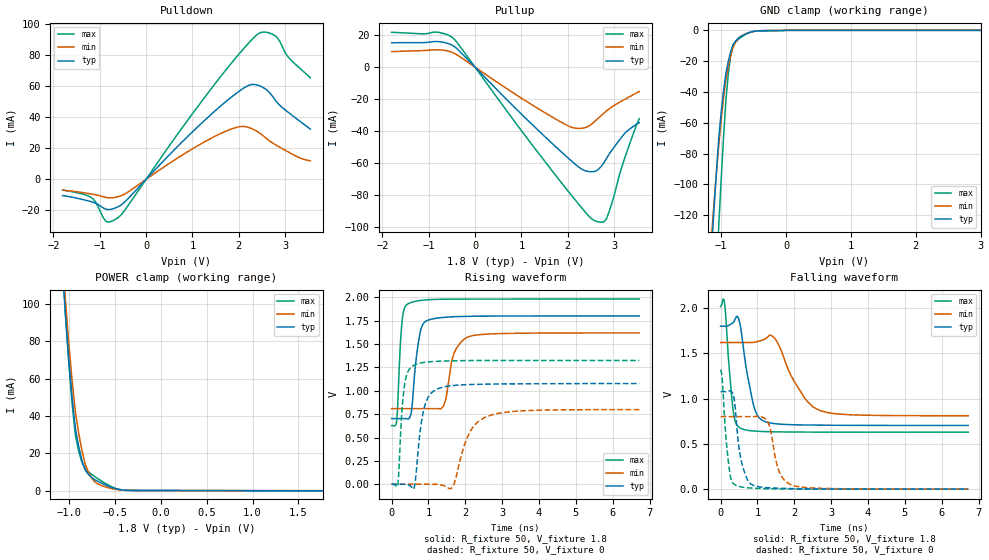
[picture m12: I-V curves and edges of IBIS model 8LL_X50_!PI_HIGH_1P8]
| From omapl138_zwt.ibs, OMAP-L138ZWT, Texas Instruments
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|   Model Cell 8LL_X50_!PI_HIGH_1P8
|BC1833DV40CTPBFZ_!PI_HIGH_1P8
[Model]   8LL_X50_!PI_HIGH_1P8
Model_type   I/O
Polarity   Non-Inverting
Enable   Active-Low
Vinl =  0.63
Vinh =  1.17
Cref =  15pF
Rref =  100.00M
Vref =  0V
Vmeas =  0.9
C_comp   2.232809p   2.073051p   2.295852p
[Model Spec]
Vinl   0.63   0.567   0.693
Vinh   1.17   1.053   1.287
[Temperature Range]   25   125   -40
[Voltage Range]   1.8   1.62   1.98
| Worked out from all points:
|   slope of the pulldown table from 0 to 0.27 V, typ, clamps not added: 31.4 ohm
|   slope of the pullup table from 0 to 0.27 V, typ, clamps not added: 33.4 ohm
|   GND clamp passes 1 mA (typ) near -0.53 V on its own axis
|   POWER clamp passes 1 mA (typ) near -0.49 V on its own axis
|   rising waveform, R_fixture 50, V_fixture 1.8: 20-80 % time 180ps typ, 264ps min, 104ps max; typ from 0.703 V to 1.8 V
|   rising waveform, R_fixture 50, V_fixture 0: 20-80 % time 231ps typ, 464ps min, 139ps max; typ from 0.003 V to 1.08 V
|   falling waveform, R_fixture 50, V_fixture 1.8: 20-80 % time 285ps typ, 638ps min, 162ps max; typ from 1.8 V to 0.705 V
|   falling waveform, R_fixture 50, V_fixture 0: 20-80 % time 222ps typ, 265ps min, 153ps max; typ from 1.08 V to 0.003 V
[POWER_clamp]
|   voltage   I(typ)   I(min)   I(max)
-1.8V     842.3mA    869.2mA    912.6mA
-1.073V   123.5mA    130.8mA    128.8mA
-1.036V   94.69mA    102.8mA    96.31mA
-1V       70.7mA     79.63mA    69.41mA
-963.6mV  50.3mA     59.44mA    47.21mA
-927.3mV  33.48mA    42.27mA    29.73mA
-854.5mV  15.97mA    21.24mA    14.89mA
-818.2mV  10.72mA    13.8mA     11.42mA
-709.1mV  5.624mA    4.312mA    7.236mA
-527.3mV  1.606mA    1.01mA     1.915mA
-381.8mV  142.3uA    117.5uA    127.8uA
1.764V    -143.5uA   -80.17uA   -225.9uA
[Pulldown]
|   voltage   I(typ)   I(min)   I(max)
-1.8V     -10.49mA   -6.992mA   -6.878mA
-1.145V   -14.77mA   -9.642mA   -12.54mA
-872.7mV  -19.18mA   -11.58mA   -26.88mA
-600mV    -17.64mA   -11.15mA   -24.61mA
1.636V    48.04mA    29.95mA    67.37mA
2.073V    58.21mA    34.18mA    83.2mA
2.291V    61.28mA    32.65mA    90.41mA
2.455V    60.33mA    29.78mA    94.55mA
2.618V    57.37mA    25.94mA    94.82mA
2.782V    51.43mA    22.55mA    92.84mA
3.055V    43.59mA    17.92mA    79.47mA
3.545V    32.43mA    11.97mA    65.61mA
[Pullup]
|   voltage   I(typ)   I(min)   I(max)
-1.8V     15.27mA    9.71mA     21.85mA
-818.2mV  16.05mA    10.88mA    21.94mA
-490.9mV  13.72mA    9.223mA    18.66mA
1.036V    -30.45mA   -20.11mA   -41.15mA
2.018V    -57.22mA   -36.91mA   -78.08mA
2.345V    -64.63mA   -38.19mA   -89.73mA
2.618V    -65.01mA   -33.11mA   -96.69mA
2.782V    -59.96mA   -28.87mA   -97.07mA
2.836V    -57.32mA   -27.51mA   -95.25mA
3V        -50.25mA   -24.09mA   -80.87mA
3.218V    -42.03mA   -20.43mA   -58.16mA
3.545V    -34.78mA   -15.26mA   -32.29mA
[GND_clamp]
|   voltage   I(typ)   I(min)   I(max)
-1.8V     -697.8mA   -553.3mA   -1.259A
-1.145V   -140.7mA   -131.7mA   -248.4mA
-1.109V   -115.2mA   -111.7mA   -203.4mA
-1.036V   -69.7mA    -74.11mA   -126mA
-963.6mV  -39.4mA    -44.23mA   -69.84mA
-927.3mV  -28.09mA   -31.91mA   -45.55mA
-890.9mV  -20.27mA   -23.39mA   -28.66mA
-854.5mV  -14.02mA   -16.45mA   -16.77mA
-818.2mV  -9.337mA   -11.08mA   -9.893mA
-672.7mV  -3.466mA   -3.226mA   -3.973mA
-18.18mV  0A         0A         0A
3.6V      0A         0A         0A
[Ramp]
| variable   typ   min   max
dV/dt_f  0.7228632/0.2988275n  0.5351467/0.6649064n  0.8824963/0.1681357n
dV/dt_r  0.6781183/0.2302543n  0.5121244/0.4699847n  0.8109243/0.1378445n
R_load = 50
[Rising Waveform]
R_fixture = 50
V_fixture = 1.8
V_fixture_min = 1.62
V_fixture_max = 1.98
|   time   V(typ)   V(min)   V(max)
0s        703.3mV    810mV      628.9mV
140ps     703.3mV    810mV      687.8mV
280ps     703mV      810mV      1.729V
450ps     698.7mV    810mV      1.93V
770ps     1.614V     810mV      1.965V
980ps     1.754V     809.9mV    1.973V
1.41ns    1.784V     837.4mV    1.978V
1.69ns    1.791V     1.399V     1.979V
2.12ns    1.796V     1.582V     1.98V
6.72ns    1.8V       1.619V     1.98V
[Rising Waveform]
R_fixture = 50
V_fixture = 0
V_fixture_min = 0
V_fixture_max = 0
|   time   V(typ)   V(min)   V(max)
0s        2.801mV    1.768mV    3.339mV
170ps     2.8mV      1.771mV    -3.328mV
340ps     2.308mV    1.768mV    1.033V
620ps     -26.36mV   1.768mV    1.276V
880ps     810.8mV    1.781mV    1.304V
1.26ns    1.023V     2.064mV    1.316V
1.62ns    1.055V     -46.3mV    1.32V
2.12ns    1.067V     557.5mV    1.323V
2.7ns     1.072V     741.4mV    1.324V
6.72ns    1.078V     799.4mV    1.324V
[Falling Waveform]
R_fixture = 50
V_fixture = 1.8
V_fixture_min = 1.62
V_fixture_max = 1.98
|   time   V(typ)   V(min)   V(max)
0s        1.8V       1.62V      2.017V
100ps     1.8V       1.62V      2.077V
340ps     1.84V      1.62V      872.8mV
540ps     1.795V     1.62V      675.2mV
910ps     905.3mV    1.622V     644.2mV
1.19ns    750.2mV    1.656V     638.1mV
1.48ns    724.8mV    1.661V     635.2mV
2.05ns    712.3mV    1.157V     632.8mV
2.7ns     708.8mV    869.1mV    632mV
6.72ns    705.4mV    812.5mV    631.5mV
[Falling Waveform]
R_fixture = 50
V_fixture = 0
V_fixture_min = 0
V_fixture_max = 0
|   time   V(typ)   V(min)   V(max)
0s        1.078V     802.6mV    1.32V
50ps      1.078V     802.6mV    1.189V
230ps     1.086V     802.6mV    246.7mV
400ps     890.1mV    802.6mV    49.24mV
570ps     300.4mV    802.6mV    26.54mV
910ps     41.77mV    802.7mV    13.71mV
1.26ns    18.92mV    762.2mV    7.961mV
1.62ns    12.26mV    167.1mV    5.443mV
1.97ns    8.7mV      42.58mV    4.522mV
6.72ns    2.861mV    3.137mV    3.973mV
